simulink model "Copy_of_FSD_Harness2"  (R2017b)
settings: Solver=FixedStepDiscrete  StartTime=0.0  StopTime=4  FixedStep=0.01  RelTol=1e-3  EnableMultiTasking=on
undefined symbols (not defined in the file): sigbuilder_block

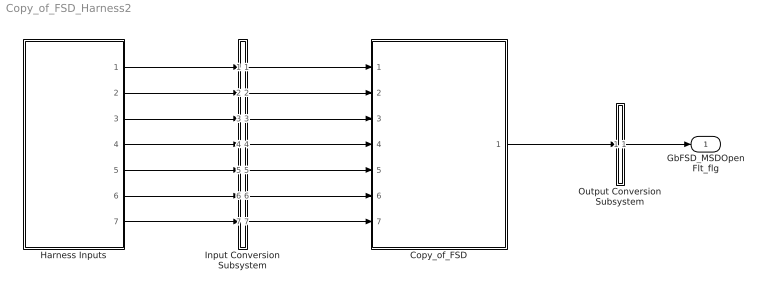
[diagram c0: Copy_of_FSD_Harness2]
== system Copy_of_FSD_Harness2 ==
  Copy_of_FSD : ModelReference  ModelNameDialog=Copy_of_FSD  SimulationMode=Normal  ModelReferenceVersion='M101C100'
  Harness Inputs : Subsystem  Tag=STV Subsys  LoadFcn=sigbuilder_block('load');  StartFcn=sigbuilder_block('start');  StopFcn=sigbuilder_block('stop');  ClipboardFcn=sigbuilder_block('clipboard');  mask(Sigbuilder block){tuvar=[0:10]}
      mask init:
      | if ~strcmp(get_param(bdroot(gcb),'SimulationStatus'),'stopped'),tuvar = sigbuilder_block('maskInit'); end
  Input Conversion Subsystem : Subsystem  Tag=__SLT_ICS__  Description=Signal spec. and routing
  Output Conversion Subsystem : Subsystem  Tag=__SLT_OCS__  Description=Signal spec. and routing
  GbFSD_MSDOpenFlt_flg : Outport  OutDataTypeStr=boolean  PortDimensions=[1]
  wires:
  Harness Inputs/1(GbHVL_HvilLFlt_flg) -> Input Conversion Subsystem/1(Inport_1)
  Harness Inputs/2(GbHDP_PackVoltVld_flg) -> Input Conversion Subsystem/2(Inport_2)
  Harness Inputs/3(GcHDP_PackVolt_V) -> Input Conversion Subsystem/3(Inport_3)
  Harness Inputs/4(GcCDP_SumCellVolt_V) -> Input Conversion Subsystem/4(Inport_4)
  Harness Inputs/5(GbCDP_SumCellVoltVld_flg) -> Input Conversion Subsystem/5(Inport_5)
  Harness Inputs/6(GbHDP_FuseVoltVld_flg) -> Input Conversion Subsystem/6(Inport_6)
  Harness Inputs/7(GcHDP_FuseVolt_V) -> Input Conversion Subsystem/7(Inport_7)
  Output Conversion Subsystem/1(Outport_1) -> GbFSD_MSDOpenFlt_flg/1
  Input Conversion Subsystem/1(Outport_1) -> Copy_of_FSD/1
  Input Conversion Subsystem/2(Outport_2) -> Copy_of_FSD/2
  Input Conversion Subsystem/3(Outport_3) -> Copy_of_FSD/3
  Input Conversion Subsystem/4(Outport_4) -> Copy_of_FSD/4
  Input Conversion Subsystem/5(Outport_5) -> Copy_of_FSD/5
  Input Conversion Subsystem/6(Outport_6) -> Copy_of_FSD/6
  Input Conversion Subsystem/7(Outport_7) -> Copy_of_FSD/7
  Copy_of_FSD/1 -> Output Conversion Subsystem/1(Inport_1)

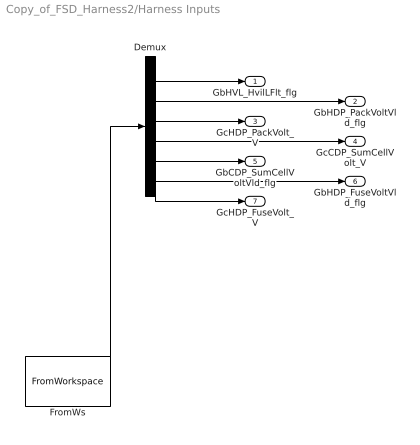
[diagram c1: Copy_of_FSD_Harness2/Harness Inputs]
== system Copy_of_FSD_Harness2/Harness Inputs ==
  Demux : Demux  Tag=STV Demux  Outputs=7
  FromWs : FromWorkspace  Tag=STV FromWs  VariableName=tuvar  SampleTime=0
  GbHVL_HvilLFlt_flg : Outport  Tag=STV Outport
  GbHDP_PackVoltVld_flg : Outport  Tag=STV Outport  Port=2
  GcHDP_PackVolt_V : Outport  Tag=STV Outport  Port=3
  GcCDP_SumCellVolt_V : Outport  Tag=STV Outport  Port=4
  GbCDP_SumCellVoltVld_flg : Outport  Tag=STV Outport  Port=5
  GbHDP_FuseVoltVld_flg : Outport  Tag=STV Outport  Port=6
  GcHDP_FuseVolt_V : Outport  Tag=STV Outport  Port=7
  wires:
  FromWs/1 -> Demux/1
  Demux/1 -> GbHVL_HvilLFlt_flg/1
  Demux/2 -> GbHDP_PackVoltVld_flg/1
  Demux/3 -> GcHDP_PackVolt_V/1
  Demux/4 -> GcCDP_SumCellVolt_V/1
  Demux/5 -> GbCDP_SumCellVoltVld_flg/1
  Demux/6 -> GbHDP_FuseVoltVld_flg/1
  Demux/7 -> GcHDP_FuseVolt_V/1

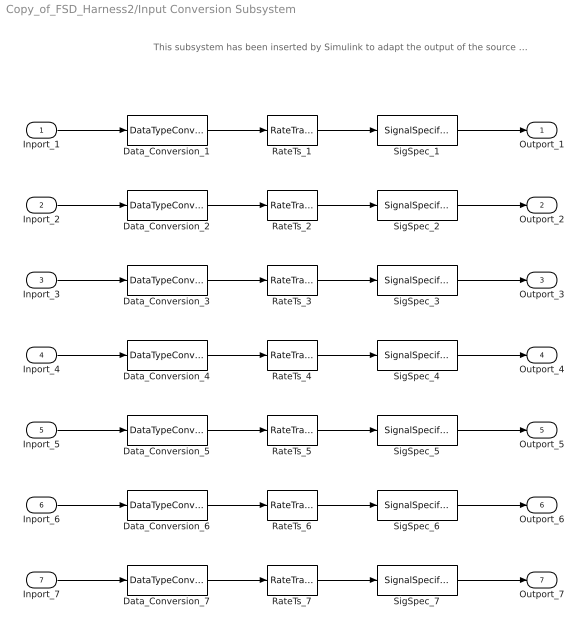
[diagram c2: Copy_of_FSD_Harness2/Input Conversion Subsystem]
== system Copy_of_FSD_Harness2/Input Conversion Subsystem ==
  note: This subsystem has been inserted by Simulink to adapt the output of the source blocks to the interface required by the harnessed component. Modifying the contents of this subsystem may result in compilation and simulation failure.
  Inport_1 : Inport
  Inport_2 : Inport  Port=2
  Inport_3 : Inport  Port=3
  Inport_4 : Inport  Port=4
  Inport_5 : Inport  Port=5
  Inport_6 : Inport  Port=6
  Inport_7 : Inport  Port=7
  Data_Conversion_{1..2,5..6} (4 alike) : DataTypeConversion  OutDataTypeStr=boolean
  Data_Conversion_3 : DataTypeConversion  OutDataTypeStr=single
  Data_Conversion_4 : DataTypeConversion  OutDataTypeStr=single
  Data_Conversion_7 : DataTypeConversion  OutDataTypeStr=single
  RateTs_{1..7} (7 alike) : RateTransition  OutPortSampleTime=0.01
  SigSpec_{1..2,5..6} (4 alike) : SignalSpecification  OutDataTypeStr=boolean  Unit=flag  Dimensions=[1]  SampleTime=0.01
  SigSpec_3 : SignalSpecification  OutDataTypeStr=single  Unit=V  Dimensions=[1]  SampleTime=0.01
  SigSpec_4 : SignalSpecification  OutDataTypeStr=single  Unit=V  Dimensions=[1]  SampleTime=0.01
  SigSpec_7 : SignalSpecification  OutDataTypeStr=single  Unit=V  Dimensions=[1]  SampleTime=0.01
  Outport_1 : Outport
  Outport_2 : Outport  Port=2
  Outport_3 : Outport  Port=3
  Outport_4 : Outport  Port=4
  Outport_5 : Outport  Port=5
  Outport_6 : Outport  Port=6
  Outport_7 : Outport  Port=7
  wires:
  SigSpec_1/1 -> Outport_1/1
  RateTs_1/1 -> SigSpec_1/1
  Data_Conversion_1/1 -> RateTs_1/1
  Inport_1/1 -> Data_Conversion_1/1
  SigSpec_2/1 -> Outport_2/1
  RateTs_2/1 -> SigSpec_2/1
  Data_Conversion_2/1 -> RateTs_2/1
  Inport_2/1 -> Data_Conversion_2/1
  SigSpec_3/1 -> Outport_3/1
  RateTs_3/1 -> SigSpec_3/1
  Data_Conversion_3/1 -> RateTs_3/1
  Inport_3/1 -> Data_Conversion_3/1
  SigSpec_4/1 -> Outport_4/1
  RateTs_4/1 -> SigSpec_4/1
  Data_Conversion_4/1 -> RateTs_4/1
  Inport_4/1 -> Data_Conversion_4/1
  SigSpec_5/1 -> Outport_5/1
  RateTs_5/1 -> SigSpec_5/1
  Data_Conversion_5/1 -> RateTs_5/1
  Inport_5/1 -> Data_Conversion_5/1
  SigSpec_6/1 -> Outport_6/1
  RateTs_6/1 -> SigSpec_6/1
  Data_Conversion_6/1 -> RateTs_6/1
  Inport_6/1 -> Data_Conversion_6/1
  SigSpec_7/1 -> Outport_7/1
  RateTs_7/1 -> SigSpec_7/1
  Data_Conversion_7/1 -> RateTs_7/1
  Inport_7/1 -> Data_Conversion_7/1

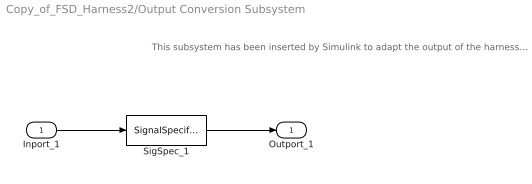
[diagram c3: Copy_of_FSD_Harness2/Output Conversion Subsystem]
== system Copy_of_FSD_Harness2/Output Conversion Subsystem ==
  note: This subsystem has been inserted by Simulink to adapt the output of the harnessed component to the interface required by the sink blocks. Modifying the contents of this subsystem may result in compilation and simulation failure.
  Inport_1 : Inport
  SigSpec_1 : SignalSpecification  OutDataTypeStr=boolean  Unit=flag  Dimensions=[1]  SampleTime=0.01
  Outport_1 : Outport
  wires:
  Inport_1/1 -> SigSpec_1/1
  SigSpec_1/1 -> Outport_1/1
